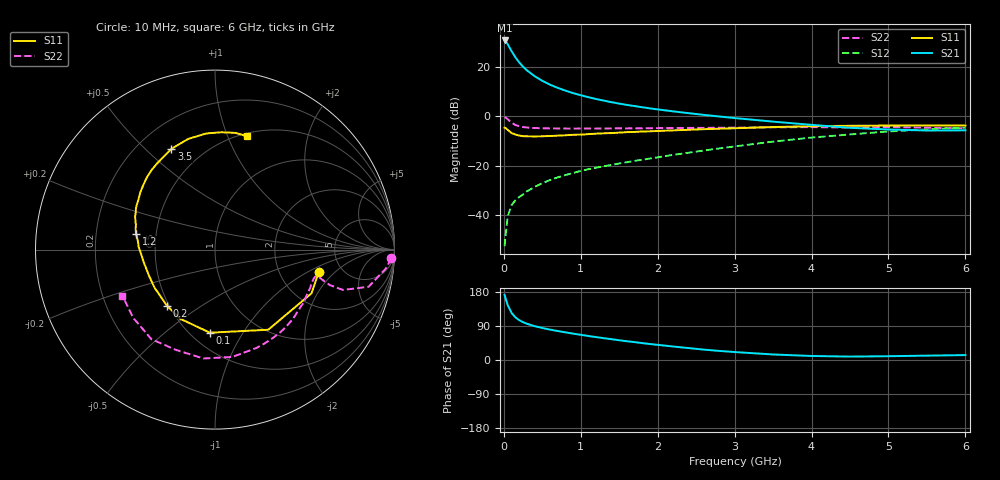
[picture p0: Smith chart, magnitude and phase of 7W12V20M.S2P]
! Infineon Technologies  Discrete & RF Semiconductors
! BFS17W
! Si NPN RF Bipolar Junction Transistor in SOT323
! VCE = 12 V  IC = 20 mA
! Common Emitter S-Parameters:  August  1999
# GHz  S  MA  R  50
!  f  S11  S21  S12  S22
! GHz  MAG  ANG  MAG  ANG  MAG  ANG  MAG  ANG
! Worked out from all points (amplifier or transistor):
!   36 points, 10 MHz to 6 GHz, reference 50 ohm
!   highest |S21| = 30.7 dB at 10 MHz (marker M1)
!   |S21| within 3 dB of that: start of sweep to 76.87 MHz
!   unconditionally stable (mu >= 1): 340.1 MHz to 1.981 GHz; 5.844 GHz to end of sweep
!   at 250 MHz: K = 0.93, MSG = 25.8 dB, |S12| = -31.5 dB
!   at 1.4 GHz: K = 1.14, MAG = 10.4 dB, |S12| = -19.6 dB
!   at 6 GHz: K = 1.01, MAG = -1.3 dB, |S12| = -4.5 dB
!   S11 on the Smith chart (normalised r, x): 10 MHz: 3.38, -1.28; 100 MHz: 0.62, -0.73; 200 MHz: 0.49, -0.37; 1.2 GHz: 0.38, +0.09; 3.5 GHz: 0.34, +0.60; 6 GHz: 0.53, +1.17
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0.01  0.5921 -12.0  34.32 172.0  0.0024 77.2  0.9842 -2.8
0.02  0.5903 -24.4  33.53 164.4  0.0037 84.6  0.9569 -6.4
0.05  0.536 -56.4  28.93 145.0  0.0095 70.3  0.8805 -13.6
0.1  0.4639 -93.5  20.91 124.5  0.0162 60.9  0.7475 -17.5
0.15  0.4313 -116.6  15.67 112.5  0.0203 59.9  0.6725 -17.2
0.2  0.4118 -130.7  12.35 105.1  0.0237 61.9  0.6347 -16.2
0.25  0.399 -140.7  10.12 99.8  0.0266 62.3  0.6117 -15.3
0.3  0.3981 -148.0  8.549 95.7  0.0308 64.3  0.5992 -14.9
0.4  0.3955 -158.5  6.517 89.3  0.0378 66.6  0.5841 -14.6
0.5  0.3981 -165.4  5.256 84.5  0.0448 68.6  0.578 -15.1
0.6  0.4037 -170.3  4.389 80.2  0.052 69.6  0.5745 -15.9
0.7  0.4096 -174.9  3.79 76.5  0.0589 70.4  0.5722 -17.1
0.9  0.4263 177.8  2.968 69.6  0.0721 71.5  0.5694 -20.0
1.1  0.4403 170.9  2.45 63.2  0.0861 72.0  0.5707 -23.5
1.2  0.4494 168.5  2.252 60.4  0.0922 72.1  0.5706 -25.4
1.6  0.4826 157.3  1.711 49.5  0.1191 73.8  0.5737 -33.5
2.2  0.5237 142.7  1.269 35.6  0.1672 75.9  0.5843 -47.2
2.8  0.5661 128.8  0.999 24.0  0.2263 74.9  0.5914 -62.2
3.5  0.6118 113.4  0.787 14.6  0.3107 70.7  0.6058 -80.7
4.5  0.6488 94.3  0.59 9.0  0.4335 58.9  0.5996 -111.0
5.5  0.6602 80.0  0.521 11.5  0.5497 45.7  0.5934 -140.3
6  0.6564 74.3  0.525 13.0  0.5963 38.9  0.5761 -153.6
